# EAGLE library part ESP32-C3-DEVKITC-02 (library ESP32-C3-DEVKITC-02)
Check availability
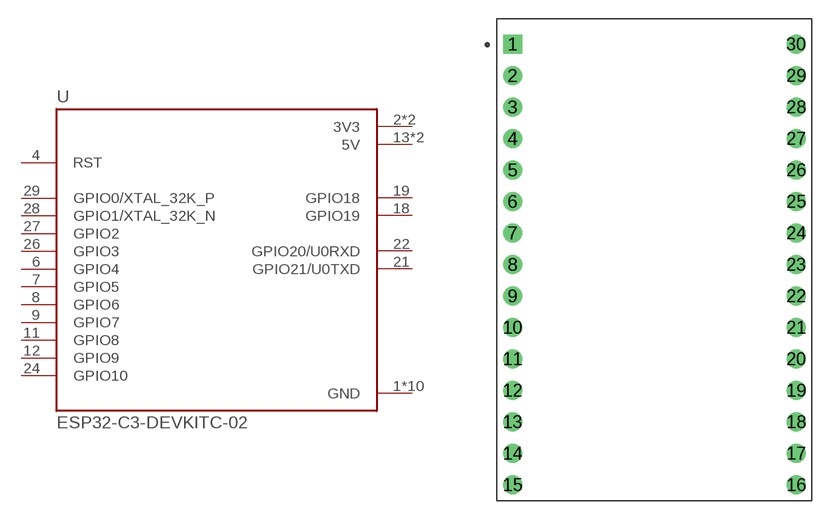
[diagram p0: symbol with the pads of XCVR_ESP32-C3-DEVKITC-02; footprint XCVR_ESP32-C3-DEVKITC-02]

Designator prefix U

## ESP32-C3-DEVKITC-02 (Availability: In Stock; Check_prices: https://www.snapeda.com/parts/ESP32-C3-DevKitC-02/Espressif+Systems/view-part/?ref=eda; Description: Development Boards & Kits - Wireless (Engineering Samples) ESP32-C3 General-Purpose Development Board, embeds ESP32-C3-WROOM-02, 4 MB Flash, with Pin Header; MF: Espressif Systems; MP: ESP32-C3-DevKitC-02; Package: None; Price: None; Purchase-URL: https://www.snapeda.com/api/url_track_click_mouser/?unipart_id=5812307&manufacturer=Espressif Systems&part_name=ESP32-C3-DevKitC-02&search_term=None; SnapEDA_Link: https://www.snapeda.com/parts/ESP32-C3-DevKitC-02/Espressif+Systems/view-part/?ref=snap)  [XCVR_ESP32-C3-DEVKITC-02]
1  GND  pwr
2  3V3  pwr
3  3V3  pwr
4  RST  in
5  GND  pwr
6  GPIO4
7  GPIO5
8  GPIO6
9  GPIO7
10  GND  pwr
11  GPIO8
12  GPIO9
13  5V  pwr
14  5V  pwr
15  GND  pwr
16  GND  pwr
17  GND  pwr
18  GPIO19
19  GPIO18
20  GND  pwr
21  GPIO21/U0TXD
22  GPIO20/U0RXD
23  GND  pwr
24  GPIO10
25  GND  pwr
26  GPIO3
27  GPIO2
28  GPIO1/XTAL_32K_N
29  GPIO0/XTAL_32K_P
30  GND  pwr

## Footprint XCVR_ESP32-C3-DEVKITC-02 (pad centres in mm)
drill 1.02 square: 1 -11.43,17.392
drill 1.02: 2 -11.43,14.852; 3 -11.43,12.312; 4 -11.43,9.772; 5 -11.43,7.232; 6 -11.43,4.692; 7 -11.43,2.152; 8 -11.43,-0.388; 9 -11.43,-2.928; 10 -11.43,-5.468; 11 -11.43,-8.008; 12 -11.43,-10.548; 13 -11.43,-13.088; 14 -11.43,-15.628; 15 -11.43,-18.168; 16 11.43,-18.168; 17 11.43,-15.628; 18 11.43,-13.088; 19 11.43,-10.548; 20 11.43,-8.008; 21 11.43,-5.468; 22 11.43,-2.928; 23 11.43,-0.388; 24 11.43,2.152; 25 11.43,4.692; 26 11.43,7.232; 27 11.43,9.772; 28 11.43,12.312; 29 11.43,14.852; 30 11.43,17.392

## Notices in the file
This work is licensed under a Creative Commons Attribution-ShareAlike 4.0 International License (CC BY-SA) with Design Exception 1.0
